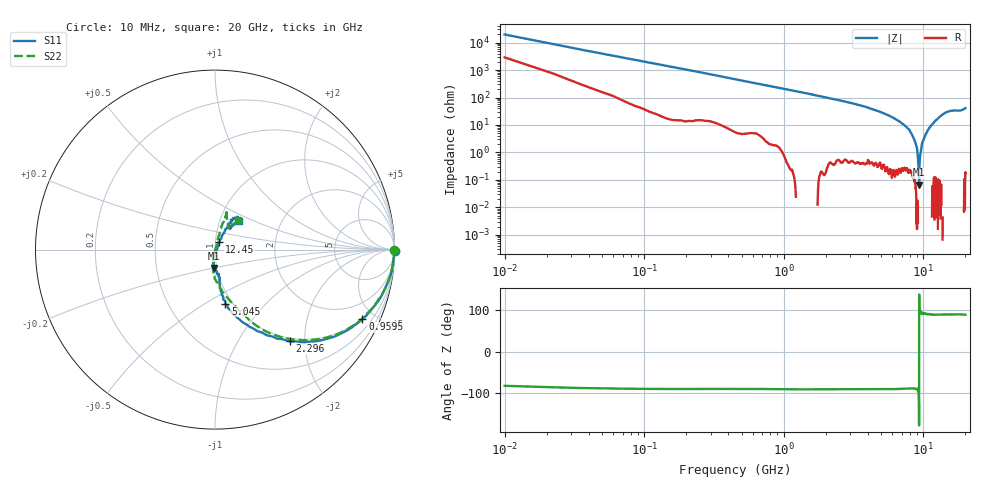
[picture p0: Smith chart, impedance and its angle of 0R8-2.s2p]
!Keysight Technologies,P5008B,MY61100088,A.16.20.02
!Date: Monday, May 27, 2024 13:32:21
!Correction: S11(C  2-Port  )
!S21(C  2-Port  )
!S12(C  2-Port  )
!S22(C  2-Port  )
!S2P File: Measurements: S11, S21, S12, S22:
# Hz S  dB  R 50
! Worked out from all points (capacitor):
!   1601 points, 10 MHz to 20 GHz, reference 50 ohm
!   read as one part in series: C = 768 fF near 110 MHz
!   lowest |Z| = 66.6 mohm at 9.318 GHz (marker M1)
!   series resonance near 9.319 GHz, so ESL is about 380 pH
!   S11 on the Smith chart (normalised r, x): 10 MHz: open; 959.5 MHz: 0.96, -4.25; 2.296 GHz: 0.94, -1.71; 5.045 GHz: 0.93, -0.62; 12.45 GHz: 1.04, +0.08; 20 GHz: 1.23, +0.41
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1e7  0.01 -0.3  -45.91 81.3  -45.81 81.4  -0.01 -0.3
1.349375e8  -0.04 -3.8  -23.69 85.4  -23.70 85.4  -0.03 -3.8
2.723688e8  -0.09 -7.8  -17.76 81.3  -17.77 81.3  -0.10 -7.5
9.59525e8  -0.84 -25.3  -7.64 64.7  -7.65 64.7  -0.83 -24.6
2.296356e9  -3.61 -50.6  -2.49 39.8  -2.50 39.9  -3.54 -48.9
3.345831e9  -5.97 -63.1  -1.25 27.5  -1.26 27.6  -6.02 -60.3
5.044981e9  -10.27 -79.2  -0.44 13.4  -0.45 13.4  -10.28 -72.9
6.681662e9  -14.37 -82.2  -0.14 4.5  -0.16 4.5  -14.34 -85.2
9.317844e9  -19.80 -93.1  -0.01 -5.8  -0.02 -5.8  -20.05 -95.8
1.0005e10  -21.81 -97.3  0.01 -8.0  0.00 -7.9  -21.90 -95.2
1.082959e10  -26.47 -94.8  0.04 -10.5  0.03 -10.5  -25.94 -101.8
1.146677e10  -34.44 -93.4  0.05 -12.5  0.04 -12.5  -33.26 -93.4
1.166667e10  -42.50 -26.5  0.04 -13.1  0.03 -13.2  -43.82 -82.8
1.176662e10  -41.46 -14.6  0.05 -13.4  0.04 -13.4  -50.05 -93.4
1.185408e10  -37.20 21.4  0.05 -13.7  0.04 -13.6  -46.65 58.7
1.199151e10  -33.12 57.3  0.04 -14.2  0.03 -14.2  -35.41 65.3
1.245378e10  -26.76 61.7  0.04 -15.6  0.03 -15.6  -27.13 71.4
1.334083e10  -18.90 61.7  0.00 -18.3  -0.01 -18.3  -18.99 75.4
1.476512e10  -13.94 60.3  -0.10 -22.8  -0.11 -22.7  -13.94 71.7
1.667666e10  -13.76 53.0  -0.11 -26.9  -0.11 -26.9  -13.75 71.5
1.861319e10  -16.92 54.2  -0.01 -32.1  -0.02 -32.0  -16.80 59.7
2e10  -13.69 50.6  -0.14 -36.8  -0.14 -36.8  -13.56 51.7
